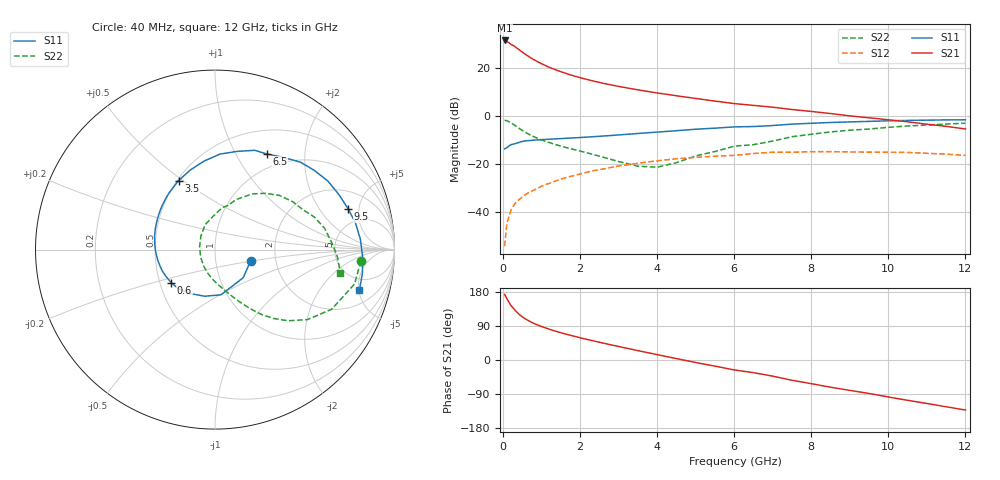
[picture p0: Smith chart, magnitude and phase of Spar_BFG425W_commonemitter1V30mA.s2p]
! Filename: 130bfg425.001
! BFG425W Field C1
! V1=8.877E-001V,V2=1.000E+000V, I1=4.808E-004A, I2=2.994E-002A
# GHz  S  MA  R 50
!  S11  S21  S12  S22
!Freq(GHz)  Mag  Ang  Mag  Ang  Mag  Ang  Mag  Ang
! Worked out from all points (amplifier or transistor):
!   44 points, 40 MHz to 12 GHz, reference 50 ohm
!   highest |S21| = 31.4 dB at 40 MHz (marker M1)
!   |S21| within 3 dB of that: start of sweep to 345.4 MHz
!   unconditionally stable (mu >= 1): start of sweep to 82.82 MHz; 791.7 MHz to end of sweep
!   at 700 MHz: K = 0.95, MSG = 27.9 dB, |S12| = -31.4 dB
!   at 2.4 GHz: K = 1.23, MAG = 15.5 dB, |S12| = -22.5 dB
!   at 12 GHz: K = 1.40, MAG = 1.7 dB, |S12| = -16.3 dB
!   S11 on the Smith chart (normalised r, x): 40 MHz: 1.48, -0.20; 600 MHz: 0.57, -0.23; 3.5 GHz: 0.51, +0.48; 6.5 GHz: 0.80, +1.35; 9.5 GHz: 3.37, +3.85; 12 GHz: 3.34, -5.05
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0.04  0.208 -18.0  37 172.8  0.002 78.6  0.815 -4.4
0.1  0.222 -44.9  35.44 161.7  0.006 79.1  0.801 -13.8
0.2  0.254 -82.4  30.89 144.6  0.011 71.9  0.73 -27.1
0.3  0.266 -102.3  27.91 132.4  0.015 67.6  0.646 -37.1
0.4  0.281 -119.4  24.27 122.2  0.018 64.5  0.568 -44.3
0.5  0.298 -132.9  21.16 113.8  0.021 62.8  0.502 -49.8
0.6  0.306 -143.0  18.59 107.2  0.024 61.9  0.45 -53.9
0.7  0.311 -151.1  16.48 101.6  0.027 60.7  0.406 -57.3
0.8  0.317 -158.1  14.78 96.6  0.029 60.3  0.372 -60.1
0.9  0.32 -163.9  13.36 92.2  0.032 59.6  0.344 -62.6
1.1  0.327 -173.9  11.15 84.6  0.038 58.2  0.299 -67.1
1.3  0.334 177.9  9.536 77.9  0.043 56.7  0.265 -71.4
1.6  0.345 167.2  7.812 69.2  0.052 53.8  0.227 -77.7
2.2  0.367 149.5  5.682 53.9  0.069 46.8  0.171 -92.7
2.8  0.395 134.1  4.431 40.0  0.086 38.5  0.126 -113.2
3.5  0.435 117.8  3.495 24.7  0.105 27.9  0.091 -151.5
4.5  0.497 97.0  2.639 3.9  0.13 11.9  0.108 137.1
6.5  0.606 61.5  1.664 -33.5  0.167 -17.6  0.255 74.0
8.5  0.736 31.2  1.128 -71.8  0.183 -53.4  0.469 40.1
9.5  0.776 17.0  0.919 -88.3  0.179 -69.1  0.538 24.4
10.5  0.812 4.1  0.76 -106.4  0.176 -86.5  0.622 11.1
12  0.836 -15.8  0.54 -132.0  0.153 -113.8  0.711 -10.5
